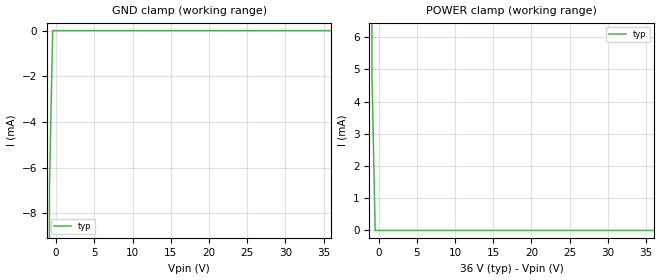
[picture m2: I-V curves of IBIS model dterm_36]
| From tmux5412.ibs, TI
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| dterm_36
[Model]   dterm_36
Model_type   Terminator
|   typ   min   max
C_comp   1.008417e-11   NA   NA
[Voltage Range]   36   NA   NA
[Temperature Range]   27   NA   NA
[Power Clamp Reference]   36   NA   NA
[GND Clamp Reference]   0   NA   NA
[GND Clamp]
|   Voltage   I(typ)   I(min)   I(max)
-5V       -2.839A    NA         NA
-1.273V   -95.92mA   NA         NA
-858.6mV  -6.733mA   NA         NA
-444.4mV  -788.2nA   NA         NA
36V       3.222nA    NA         NA
[POWER Clamp]
|   Voltage   I(typ)   I(min)   I(max)
-5V       2.61A      NA         NA
-1.273V   85.35mA    NA         NA
-858.6mV  4.769mA    NA         NA
-444.4mV  101.5nA    NA         NA
36V       -1.437nA   NA         NA
